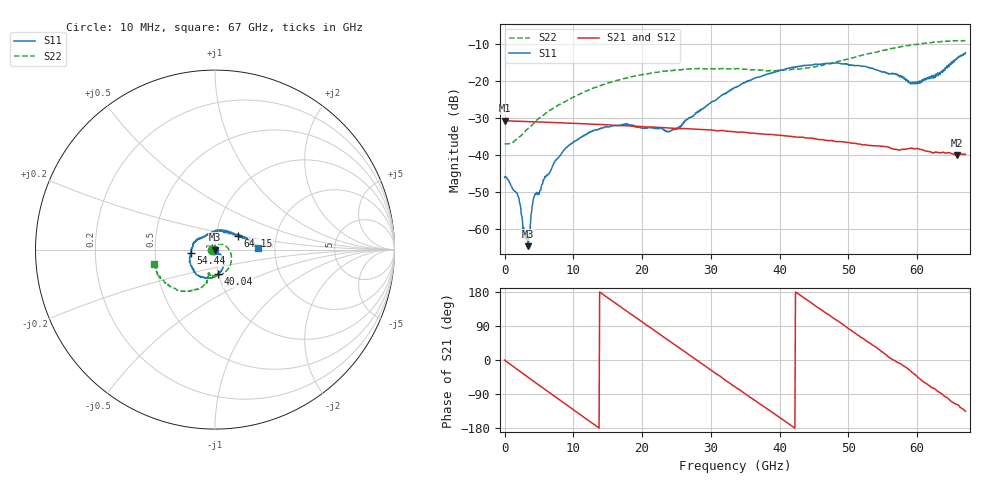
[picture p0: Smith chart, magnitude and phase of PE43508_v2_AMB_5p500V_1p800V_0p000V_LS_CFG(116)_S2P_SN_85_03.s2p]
!Keysight Technologies,N5227A,US51270237,A.10.43.00
!Date: Wednesday, August 22, 2018 17:18:48
!Correction: S11(Full 2 Port(1,3))
!S31(Full 2 Port(1,3))
!S13(Full 2 Port(1,3))
!S33(Full 2 Port(1,3))
!S2P File: Measurements: S11, S31, S13, S33:
# Hz S  dB  R 50
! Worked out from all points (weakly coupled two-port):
!   801 points, 10 MHz to 67 GHz, reference 50 ohm
!   highest |S21| = -30.76 dB at 10 MHz (marker M1); lowest = -40.0 dB at 65.83 GHz (marker M2)
!   lowest |S11| = -64.7 dB at 3.443 GHz (marker M3), VSWR 1.00, Z = 50 + j0.0374 ohm
!   |S11| at or under -10 dB: start of sweep to end of sweep
!   |S22| runs from -37.1 to -9.1 dB; largest |S21 - S12| = 0.00018
!   S11 on the Smith chart (normalised r, x): 10 MHz: 0.99, -0.00; 40.04 GHz: 1.00, -0.28; 54.44 GHz: 0.76, -0.03; 64.15 GHz: 1.27, +0.19; 67 GHz: 1.63, +0.03
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1e7  -46.12 -176.5  -30.76 -0.3  -30.77 -0.2  -37.05 -179.7
1.852225e9  -50.41 155.7  -30.91 -25.0  -30.91 -25.0  -35.54 124.0
2.940812e9  -62.48 107.3  -30.98 -39.4  -30.98 -39.4  -33.74 99.4
3.192025e9  -63.10 80.4  -31.00 -42.7  -31.00 -42.7  -33.26 95.0
3.443238e9  -64.65 39.6  -31.02 -46.0  -31.02 -46.0  -32.86 90.9
4.113138e9  -52.78 -14.9  -31.06 -54.7  -31.06 -54.7  -31.75 80.1
4.448088e9  -50.45 -5.8  -31.07 -59.1  -31.08 -59.1  -31.06 75.5
7.546375e9  -41.37 -44.7  -31.30 -99.4  -31.30 -99.4  -26.88 43.2
1.123082e10  -35.02 -65.4  -31.57 -147.1  -31.58 -147.1  -23.31 10.8
1.74274e10  -31.75 -88.3  -32.11 133.4  -32.10 133.4  -19.36 -31.2
2.236791e10  -32.82 -84.2  -32.60 70.3  -32.59 70.2  -17.64 -58.3
2.513125e10  -32.62 -64.9  -32.87 35.5  -32.86 35.4  -17.01 -70.8
3.3505e10  -21.84 -55.4  -33.80 -71.1  -33.79 -71.1  -16.73 -98.8
4.003652e10  -17.25 -82.7  -34.70 -152.3  -34.68 -152.3  -17.11 -105.3
4.472582e10  -15.72 -106.9  -35.54 148.9  -35.52 149.0  -16.39 -103.3
4.841028e10  -15.18 -127.0  -36.42 103.6  -36.41 103.5  -14.84 -104.1
5.443938e10  -17.30 -172.1  -37.57 27.9  -37.55 27.5  -12.08 -116.3
5.586291e10  -18.20 171.4  -37.96 7.5  -37.95 7.2  -11.42 -120.8
5.979858e10  -20.37 113.1  -38.26 -40.3  -38.28 -40.6  -10.20 -134.6
6.415292e10  -16.67 30.2  -39.56 -97.2  -39.58 -97.5  -9.31 -153.1
6.582768e10  -13.86 14.5  -40.02 -117.9  -40.07 -118.2  -9.18 -160.2
6.7e10  -12.38 1.8  -39.88 -135.3  -39.95 -135.2  -9.12 -166.7
